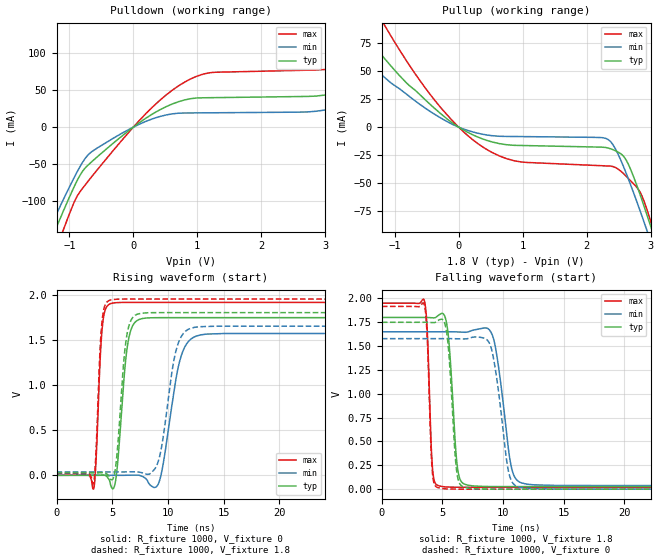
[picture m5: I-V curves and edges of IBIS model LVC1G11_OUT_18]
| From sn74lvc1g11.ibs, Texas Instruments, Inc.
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[Model]   LVC1G11_OUT_18
Model_type  Output
Vref =   0
Rref =   1000
Cref =   30p
Vmeas =   0.9
| variable   typ   min   max
C_comp   8.96pF   6.63pF   13.10pF
| C_pullup   8.25pF   6.63pF   8.86pF
| C_pulldown   9.66pF   6.75pF   13.10pF
[Temperature Range]   40   100   -40
| Ambient temperature   25   85   -40
[Voltage range]   1.8   1.65   1.95
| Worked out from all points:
|   slope of the pulldown table from 0 to 0.27 V, typ, clamps not added: 16.6 ohm
|   slope of the pullup table from 0 to 0.27 V, typ, clamps not added: 33.2 ohm
|   rising waveform, R_fixture 1000, V_fixture 0: 20-80 % time 697ps typ, 1.23ns min, 407ps max; typ from 0 V to 1.74 V
|   falling waveform, R_fixture 1000, V_fixture 1.8: 20-80 % time 520ps typ, 933ps min, 310ps max; typ from 1.8 V to 0.027 V
|   rising waveform, R_fixture 1000, V_fixture 1.8: 20-80 % time 663ps typ, 1.14ns min, 396ps max; typ from 0.027 V to 1.8 V
|   falling waveform, R_fixture 1000, V_fixture 0: 20-80 % time 510ps typ, 921ps min, 306ps max; typ from 1.75 V to 0 V
[Pulldown]
| LVC1G11_OUT_18
|   Voltage   I(typ)   I(min)   I(max)
-5.5V     -1.024A    -932.8mA   -1.173A
-1.44V    -185.2mA   -162.4mA   -222.4mA
-1.105V   -116mA     -100.2mA   -142mA
-645mV    -46.52mA   -32.98mA   -66.62mA
805mV     36.94mA    19.18mA    61.21mA
3.215V    47.58mA    27.05mA    81.88mA
4.145V    78.53mA    21.52mA    125.4mA
4.31V     68.9mA     21.59mA    136.1mA
4.47V     45.47mA    21.68mA    146.3mA
4.7V      44.48mA    21.82mA    139.5mA
5.01V     44.71mA    22mA       83.15mA
11V       50.72mA    25.33mA    93.05mA
[Pullup]
| LVC1G11_OUT_18
|   Voltage   I(typ)   I(min)   I(max)
-5.5V     476.4mA    372.8mA    667mA
-1.985V   124.4mA    93.02mA    180.5mA
-1.605V   93.94mA    69.4mA     137.6mA
-1.145V   60.57mA    43.87mA    89.95mA
-350mV    15.5mA     10.6mA     22.36mA
440mV     -11.85mA   -7.028mA   -20.01mA
2.34V     -18.76mA   -11.2mA    -34.79mA
2.625V    -30.23mA   -42.31mA   -44.38mA
2.93V     -76.38mA   -90.38mA   -71.68mA
3.03V     -93.86mA   -107.1mA   -89.69mA
3.115V    -109.1mA   -121.5mA   -106mA
11V       -1.709A    -1.61A     -1.886A
[Ramp]
| LVC1G11_OUT_18
| variable   typ   min   max
dV/dt_r   1.14/7.44E-10   1.02/1.31E-09   1.24/4.37E-10
dV/dt_f   1.09/5.40E-10   0.99/9.65E-10   1.18/3.28E-10
R_load = 1000
[Rising Waveform]
| LVC1G11_OUT_18
R_fixture =   1000
C_fixture =   0
L_fixture =   0
V_fixture =   0
V_fixture_min = 0
V_fixture_max = 0
|   Time   V(typ)   V(min)   V(max)
0s        112.7pV    7.663nV    2.84nV
3.335ns   -46.98uV   2.162uV    -150.4mV
4.095ns   2.55mV     -27.77nV   1.62V
4.86ns    -108mV     -39.6uV    1.9V
6.425ns   1.475V     1.246mV    1.913V
7.425ns   1.725V     391.2uV    1.913V
9.17ns    1.744V     -88.06mV   1.913V
11.05ns   1.744V     1.256V     1.913V
12.57ns   1.744V     1.542V     1.913V
43ns      1.744V     1.569V     1.913V
[Falling Waveform]
| LVC1G11_OUT_18
R_fixture =   1000
C_fixture =   0
L_fixture =   0
V_fixture =   1.8
V_fixture_min = 1.65
V_fixture_max = 1.95
|   Time   V(typ)   V(min)   V(max)
0s        1.8V       1.65V      1.95V
3.505ns   1.8V       1.65V      1.978V
4.165ns   1.797V     1.65V      243.9mV
4.625ns   1.818V     1.65V      39.2mV
5.38ns    1.714V     1.65V      22.71mV
6.21ns    255.2mV    1.648V     20.17mV
6.885ns   49.68mV    1.644V     19.83mV
9.135ns   27.47mV    1.609V     19.73mV
11.52ns   27mV       65.71mV    19.73mV
43ns      26.97mV    37.14mV    19.72mV
[Rising Waveform]
| LVC1G11_OUT_18
R_fixture =   1000
C_fixture =   0
L_fixture =   0
V_fixture =   1.8
V_fixture_min = 1.65
V_fixture_max = 1.95
|   Time   V(typ)   V(min)   V(max)
0s        26.95mV    37.1mV     19.71mV
3.32ns    26.91mV    37.1mV     -86.98mV
4.055ns   29.21mV    37.1mV     1.663V
4.78ns    -22.29mV   37.07mV    1.937V
5.335ns   119.7mV    37.09mV    1.948V
6.31ns    1.546V     37.91mV    1.95V
7.235ns   1.782V     38.66mV    1.95V
9.08ns    1.8V       133.2mV    1.95V
12.03ns   1.8V       1.625V     1.95V
43ns      1.8V       1.65V      1.95V
[Falling Waveform]
| LVC1G11_OUT_18
R_fixture =   1000
C_fixture =   0
L_fixture =   0
V_fixture =   0
V_fixture_min = 0
V_fixture_max = 0
|   Time   V(typ)   V(min)   V(max)
0s        1.749V     1.578V     1.916V
3.495ns   1.75V      1.578V     1.938V
4.14ns    1.747V     1.578V     227.6mV
4.605ns   1.766V     1.578V     17.48mV
5.35ns    1.645V     1.578V     2.808mV
6.14ns    226.9mV    1.577V     464.9uV
6.78ns    21.25mV    1.575V     129.9uV
8.955ns   520.9uV    1.508V     19.57uV
11.22ns   42.53uV    25.22mV    17.07uV
43ns      16.21uV    31.31uV    8.958uV
